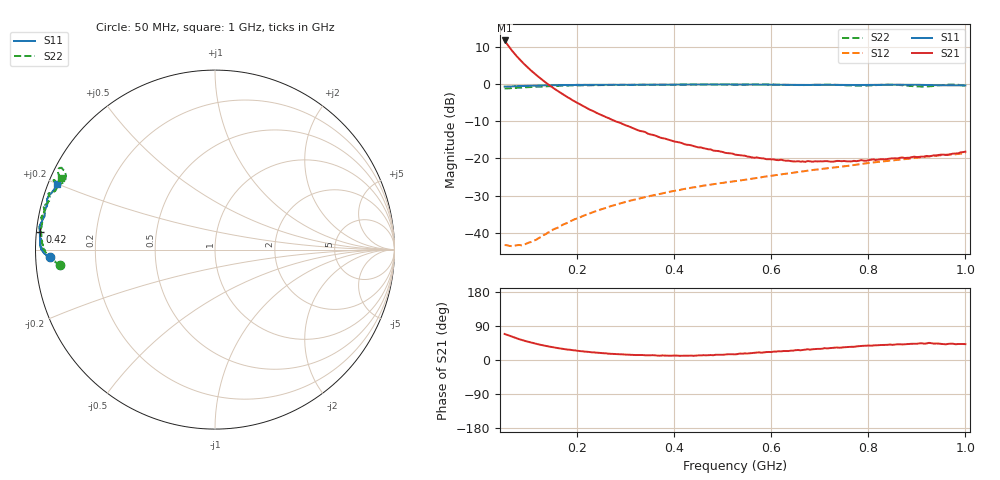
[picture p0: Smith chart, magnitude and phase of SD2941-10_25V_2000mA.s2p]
!Agilent Technologies,E8358A,US42080673,A.04.86
!Agilent E8358A: A.04.86
!Date: Friday, June 09, 2006 14:46:01
!Correction: S11(Full 2 Port SOLT,1,2) S21(Full 2 Port SOLT,1,2) S12(Full 2 Port SOLT,1,2) S22(Full 2 Port SOLT,1,2)
!S2P File: Measurements: S11, S21, S12, S22:
# Hz S  MA  R 50
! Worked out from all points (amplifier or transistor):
!   191 points, 50 MHz to 1 GHz, reference 50 ohm
!   highest |S21| = 11.7 dB at 50 MHz (marker M1)
!   |S21| within 3 dB of that: start of sweep to 66.99 MHz
!   unconditionally stable (mu >= 1): 753.8 MHz to 815.8 MHz; 874.7 MHz to 957.8 MHz; 990.7 MHz to end of sweep
!   at 205 MHz: K = 0.49, MSG = 15.2 dB, |S12| = -35.9 dB
!   at 525 MHz: K = 0.46, MSG = 3.6 dB, |S12| = -26.1 dB
!   at 1 GHz: K = 1.09, MAG = -1.6 dB, |S12| = -18.6 dB
!   S11 on the Smith chart (normalised r, x): 50 MHz: 0.04, -0.02; 420 MHz: 0.01, +0.05; 1 GHz: 0.02, +0.20
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5e7  0.9209 -177.6  3.832 68.7  0.006866 19.6  0.8672 -174.3
5.5e7  0.9245 -177.4  3.434 66.4  0.006839 21.1  0.8723 -174.4
6e7  0.9261 -177.7  3.103 63.8  0.006688 24.1  0.8737 -174.7
6.5e7  0.9256 -177.6  2.811 61.4  0.006641 26.7  0.8798 -174.8
7e7  0.932 -177.8  2.571 59.3  0.006734 29.8  0.8838 -175.2
7.5e7  0.9313 -177.9  2.353 57.1  0.00683 33.0  0.8858 -175.2
8.5e7  0.9383 -178.1  2.006 53.0  0.006815 38.8  0.8924 -175.7
1e8  0.9437 -178.4  1.606 47.6  0.007427 49.2  0.9054 -176.2
1.2e8  0.9508 -178.7  1.244 41.2  0.00851 60.3  0.9184 -176.9
1.4e8  0.9575 -179.3  0.9838 35.8  0.01016 66.2  0.9309 -178.0
1.75e8  0.9681 179.9  0.6935 28.4  0.01328 73.7  0.9475 -179.4
2.1e8  0.9703 179.1  0.5112 23.0  0.01674 76.7  0.9587 179.1
2.8e8  0.9729 177.1  0.3127 15.7  0.02403 78.3  0.9669 176.1
3.7e8  0.9772 175.5  0.1913 11.4  0.03333 77.4  0.9775 173.0
4.2e8  0.9808 174.1  0.1559 11.0  0.0389 75.8  0.9759 170.7
5.25e8  0.9835 172.1  0.1125 14.9  0.04948 73.5  0.974 167.7
6.85e8  0.9717 168.0  0.09041 28.4  0.06971 69.4  0.9705 162.1
7.85e8  0.9682 165.2  0.09486 37.1  0.08401 66.8  0.9449 158.7
8.45e8  0.9749 163.6  0.09976 40.9  0.09297 64.8  0.9765 156.8
9e8  0.9741 162.0  0.104 42.9  0.1022 62.9  0.926 156.3
9.55e8  0.9582 159.8  0.1125 42.0  0.111 60.8  0.968 151.9
1e9  0.9548 157.4  0.1233 41.9  0.1177 56.9  0.9445 155.1
